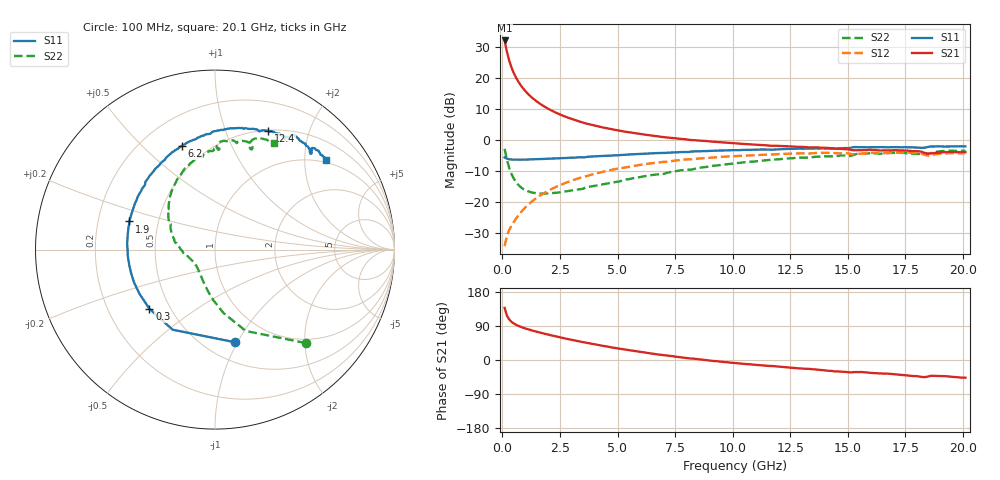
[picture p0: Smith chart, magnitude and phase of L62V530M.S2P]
!  Infineon Technologies AG
! BFR380L3 , PF131585-7, No.6, Th 09.10.01, soldered on pcb-board, measured with PP GSG850
!  Vce=2.5 V,  Ic=30.0 mA
! Common Emitter S-Parameters:  15. November 2001
#  GHz  S  MA  R  50
! f  S11  S21  S12  S22
! GHz  Mag  Ang  Mag  Ang  Mag  Ang  Mag  Ang
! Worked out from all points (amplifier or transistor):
!   201 points, 100 MHz to 20.1 GHz, reference 50 ohm
!   highest |S21| = 32.3 dB at 100 MHz (marker M1)
!   |S21| within 3 dB of that: start of sweep to 182 MHz
!   unconditionally stable (mu >= 1): 1.184 GHz to 4.356 GHz
!   at 3.4 GHz: K = 1.02, MAG = 8.2 dB, |S12| = -12.1 dB
!   at 10.1 GHz: K = 0.96, MSG = 2.0 dB, |S12| = -5.1 dB
!   at 20.1 GHz: K = 0.99, MSG = 0.2 dB, |S12| = -4.2 dB
!   S11 on the Smith chart (normalised r, x): 100 MHz: 0.68, -0.98; 300 MHz: 0.38, -0.33; 1.9 GHz: 0.34, +0.14; 6.2 GHz: 0.36, +0.66; 12.4 GHz: 0.51, +1.42; 20.1 GHz: 0.93, +2.53
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0.1  0.5287 -77.7  41.1 137.5  0.01938 60.9  0.7263 -45.8
0.2  0.5049 -117.9  26.97 117.0  0.02868 56.0  0.4848 -69.3
0.3  0.4921 -137.9  19.38 107.0  0.03551 57.0  0.3564 -82.4
0.4  0.4876 -149.9  14.99 100.7  0.04157 58.7  0.2838 -91.6
0.5  0.4867 -158.1  12.18 96.3  0.04783 61.1  0.2391 -98.8
0.6  0.4854 -164.1  10.23 92.9  0.05463 62.9  0.2097 -104.8
0.7  0.4853 -168.8  8.832 90.0  0.06115 64.1  0.1891 -110.2
0.8  0.4858 -172.7  7.756 87.5  0.06807 65.2  0.1746 -114.8
1  0.4867 -179.0  6.253 83.3  0.08206 66.3  0.1559 -122.8
1.2  0.4907 175.8  5.24 79.5  0.09616 66.6  0.1458 -129.5
1.5  0.4944 169.2  4.228 74.4  0.1175 66.3  0.1385 -137.7
1.9  0.5022 161.8  3.378 68.3  0.146 64.9  0.1373 -146.5
2.6  0.514 150.6  2.521 58.5  0.1945 61.4  0.1461 -158.6
3.5  0.5304 137.8  1.932 47.1  0.2553 55.6  0.164 -170.0
4.8  0.5683 122.2  1.497 32.7  0.335 46.7  0.208 173.2
6.2  0.607 107.8  1.233 19.4  0.411 36.8  0.2631 157.8
6.8  0.6209 102.2  1.15 14.2  0.4396 32.4  0.2827 151.1
10.1  0.692 77.9  0.8888 -7.9  0.5551 10.9  0.4241 122.4
12.4  0.7252 66.0  0.7993 -19.6  0.607 -3.1  0.5068 104.0
13.5  0.734 60.7  0.7687 -24.6  0.6181 -9.4  0.5339 96.8
16.8  0.771 48.5  0.6884 -36.3  0.6252 -25.1  0.6217 76.7
20.1  0.7947 38.9  0.6422 -46.7  0.6193 -38.6  0.6776 61.0
